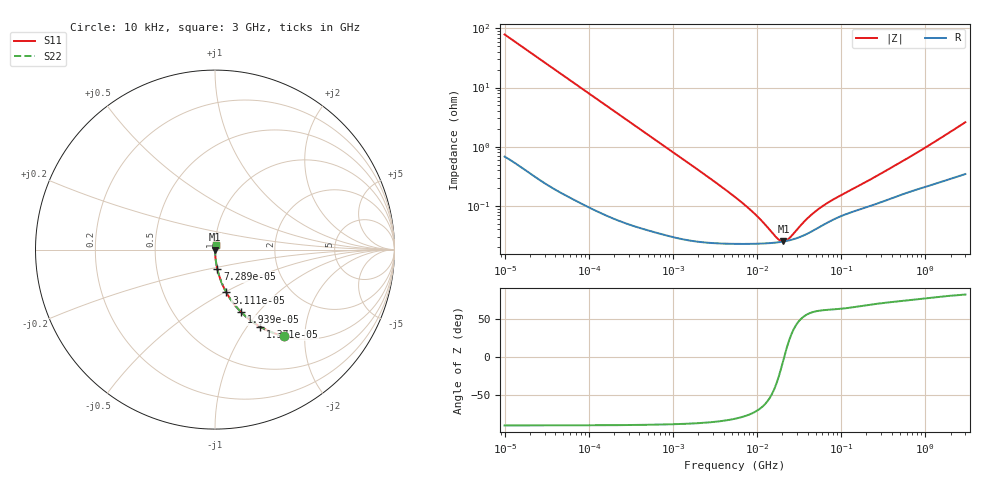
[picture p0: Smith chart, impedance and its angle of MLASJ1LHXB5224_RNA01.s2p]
! MLASJ1LHXB5224_RNA01  S-PARAMETER MODEL  ( Standard Model )
! Model Generated by TAIYO YUDEN Corporation (http://www.ty-top.com)
! Version 1.0
! TAIYO YUDEN Control No. 220601
! Copyright(c) 2015 TAIYO YUDEN CO.,LTD. All Rights Reserved.
! Product Description (link to TY-COMPAS)
! https://ds.yuden.co.jp/TYCOMPAS/or/detail?pn=MLASJ1LHXB5224MRNA01&u=M
! Products Name : Multilayer Ceramic Capacitors
! Characteristics :
!  Capacitance : 0.22 [uF] , Rated Voltage : 6.3 [V] , TCC : X5R
!  Case Size : 1.0 x 0.5 / 0.039 x 0.02 [mm/inch] , Thickness : 0.13 / 0.005 [mm/inch]
!  (Conditions: Temperature = 25 [degC] , DC Bias Voltage = 0 [V])
! External Node Assignments :
!  1  o---| |---o  2
! GND o---------o GND
! Frequency Range : 10kHz  -  3GHz  [ 401 STEP ]
# MHZ S RI R 50
! Freq[MHz].  S11 Real  S11 Imag  S21 Real  S21 Imag  S12 Real  S12 Imag  S22 Real  S22 Imag
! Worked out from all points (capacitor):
!   401 points, 10 kHz to 3 GHz, reference 50 ohm
!   read as one part in series: C = 201 nF near 10.65 kHz
!   lowest |Z| = 25 mohm at 20.59 MHz (marker M1)
!   series resonance near 21.01 MHz, so ESL is about 290 pH
!   S11 on the Smith chart (normalised r, x): 10 kHz: 1.01, -1.58; 13.71 kHz: 1.01, -1.16; 19.39 kHz: 1.01, -0.82; 31.11 kHz: 1.00, -0.51; 72.89 kHz: 1.00, -0.22; 3 GHz: 1.01, +0.05
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0.01  0.3854 -0.4824  0.6146 0.4824  0.6146 0.4824  0.3854 -0.4824
0.013707  0.2522 -0.4298  0.7478 0.4298  0.7478 0.4298  0.2522 -0.4298
0.019389  0.1457 -0.3484  0.8543 0.3484  0.8543 0.3484  0.1457 -0.3484
0.031113  0.0633 -0.2389  0.9367 0.2389  0.9367 0.2389  0.0633 -0.2389
0.046876  0.0296 -0.1647  0.9704 0.1647  0.9704 0.1647  0.0296 -0.1647
0.072886  0.013 -0.1081  0.987 0.1081  0.987 0.1081  0.013 -0.1081
0.082683  0.0103 -0.0956  0.9897 0.0956  0.9897 0.0956  0.0103 -0.0956
0.199902  0.00221 -0.0401  0.9978 0.0401  0.9978 0.0401  0.00221 -0.0401
0.683653  0.000481 -0.0118  0.9995 0.0118  0.9995 0.0118  0.000481 -0.0118
2.570001  0.000248 -0.00313  0.9998 0.00313  0.9998 0.00313  0.000248 -0.00313
5.477226  0.000229 -0.00139  0.9998 0.00139  0.9998 0.00139  0.000229 -0.00139
9.97066  0.000229 -0.000636  0.9998 0.000636  0.9998 0.000636  0.000229 -0.000636
17.5871  0.000241 -0.000139  0.9998 0.000139  0.9998 0.000139  0.000241 -0.000139
19.33182  0.000246 -6.49e-05  0.9998 6.49e-05  0.9998 6.49e-05  0.000246 -6.49e-05
20.5901  0.000249 -1.57e-05  0.9998 1.57e-05  0.9998 1.57e-05  0.000249 -1.57e-05
24.10585  0.000261 0.000107  0.9997 -0.000107  0.9997 -0.000107  0.000261 0.000107
35.19136  0.000312 0.00041  0.9997 -0.00041  0.9997 -0.00041  0.000312 0.00041
45.28751  0.000373 0.000622  0.9996 -0.000622  0.9996 -0.000622  0.000373 0.000622
58.28018  0.000458 0.000842  0.9995 -0.000842  0.9995 -0.000842  0.000458 0.000842
77.4027  0.000569 0.0011  0.9994 -0.0011  0.9994 -0.0011  0.000569 0.0011
374.4521  0.00131 0.00403  0.9987 -0.00403  0.9987 -0.00403  0.00131 0.00403
3000  0.00409 0.0255  0.9959 -0.0255  0.9959 -0.0255  0.00409 0.0255
